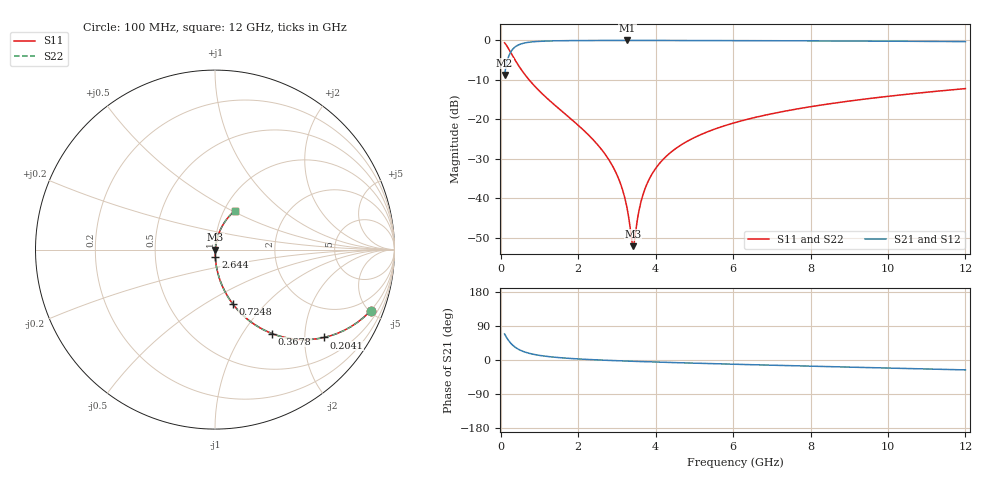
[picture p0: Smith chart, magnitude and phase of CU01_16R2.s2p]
! S-parameter model data by Modelithics Inc. support@modelithics.com 813-866-6335 Tampa FL USA
! S-Parameter data specifications:
! Substrate: 20-mil Rogers, substrate thickness, H=0.508mm, Dielectric constant, Er=3.75
! PCB Mounting Pad Footprint: Pad width, PadW=0.35mm , Pad length, PadL=0.30mm , Pad gap, PadG (edge-to-edge)=0.25mm , Reference planes=0.85mm apart
! Created Tue May  8 14:01:25 2018
# hz S ma R 50
! 2 Port Network Data from SP1.SP block
! freq  magS11  angS11  magS21  angS21  magS12  angS12  magS22  angS22
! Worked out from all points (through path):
!   801 points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, 100 MHz to 12 GHz, reference 50 ohm
!   highest |S21| = -0.02 dB at 3.268 GHz (marker M1); lowest = -8.8 dB at 100 MHz (marker M2)
!   group delay of S21, straight-line fit = 10.5 ps
!   lowest |S11| = -52.2 dB at 3.417 GHz (marker M3), VSWR 1.00, Z = 50.2 - j0.026 ohm
!   |S11| at or under -10 dB: 732 MHz to end of sweep
!   |S22| runs from -52.2 to -0.6 dB; largest |S21 - S12| = 0
!   S11 on the Smith chart (normalised r, x): 100 MHz: 0.99, -5.09; 204.1 MHz: 0.99, -2.49; 367.8 MHz: 0.99, -1.37; 724.8 MHz: 0.99, -0.67; 2.644 GHz: 1.00, -0.08; 12 GHz: 1.12, +0.52
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1e8  0.9312 -21.4  0.364 68.5  0.364 68.5  0.9312 -21.4
2.04125e8  0.7805 -38.8  0.6245 51.1  0.6245 51.1  0.7805 -38.8
3.6775e8  0.5665 -55.8  0.8231 34.1  0.8231 34.1  0.5665 -55.8
5.165e8  0.4355 -64.6  0.899 25.3  0.899 25.3  0.4355 -64.6
7.2475e8  0.3193 -71.9  0.9463 17.9  0.9463 17.9  0.3193 -71.9
1.26025e9  0.1727 -80.8  0.9833 8.7  0.9833 8.7  0.1727 -80.8
2.09325e9  0.07626 -86.2  0.995 2.3  0.995 2.3  0.07626 -86.2
2.643625e9  0.03902 -87.2  0.997 -0.4  0.997 -0.4  0.03902 -87.2
3.030375e9  0.01831 -84.7  0.9975 -2.0  0.9975 -2.0  0.01831 -84.7
3.16425e9  0.01189 -81.0  0.9975 -2.5  0.9975 -2.5  0.01189 -81.0
3.268375e9  0.007205 -73.3  0.9975 -2.9  0.9975 -2.9  0.007205 -73.3
3.3725e9  0.003212 -43.7  0.9975 -3.3  0.9975 -3.3  0.003212 -43.7
3.417125e9  0.00246 -6.0  0.9975 -3.4  0.9975 -3.4  0.00246 -6.0
3.46175e9  0.003076 33.0  0.9975 -3.6  0.9975 -3.6  0.003076 33.0
3.58075e9  0.007348 66.1  0.9974 -4.0  0.9974 -4.0  0.007348 66.1
3.69975e9  0.01209 73.5  0.9973 -4.4  0.9973 -4.4  0.01209 73.5
4.071625e9  0.02647 78.7  0.9969 -5.6  0.9969 -5.6  0.02647 78.7
4.83025e9  0.05302 79.1  0.9957 -7.9  0.9957 -7.9  0.05302 79.1
6.05e9  0.09065 76.8  0.9927 -11.3  0.9927 -11.3  0.09065 76.8
8.04325e9  0.1453 72.2  0.9857 -16.4  0.9857 -16.4  0.1453 72.2
1.002162e10  0.1958 67.5  0.9765 -21.3  0.9765 -21.3  0.1958 67.5
1.2e10  0.2447 62.8  0.9648 -26.1  0.9648 -26.1  0.2447 62.8
